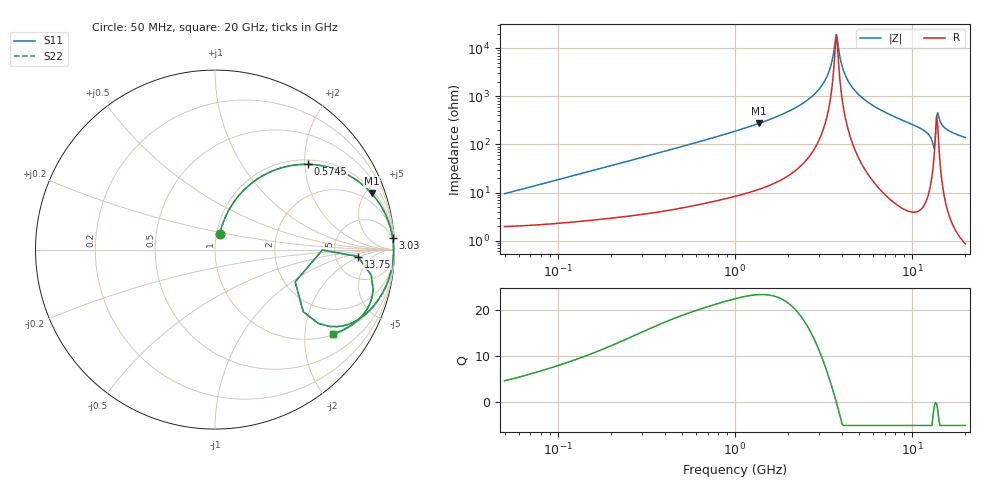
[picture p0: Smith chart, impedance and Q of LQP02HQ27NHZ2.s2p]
!Murata Part Number: LQP02HQ27NHZ2
!These Parameters are Measured in Series Mode Connection
!  o--[Z]--o
!Port1  Port2
!  o-------o
!Freq. Start=50[MHz] Stop=20[GHz], 401[Steps]
# Hz S RI R 50
!Freq.(Hz) S11(Real) S11(Imag) S21(Real) S21(Imag) S12(Real) S12(Imag) S22(Real) S22(Imag)
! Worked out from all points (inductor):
!   401 points, 50 MHz to 20 GHz, reference 50 ohm
!   read as one part in series: L = 29.4 nH near 51.52 MHz
!   highest Q = 23.4 at 1.37 GHz (marker M1), where L = 31.9 nH
!   self-resonance near 3.736 GHz
!   S11 on the Smith chart (normalised r, x): 50 MHz: 1.04, +0.19; 574.5 MHz: 1.11, +2.08; 3.03 GHz: 4, +30; 13.75 GHz: 8.53, -1.84; 20 GHz: 1.02, -2.77
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5e7  0.0273 0.0884  0.9727 -0.0884  0.9727 -0.0884  0.0273 0.0884
1.364002e8  0.079 0.2235  0.921 -0.2235  0.921 -0.2235  0.079 0.2235
3.721004e8  0.3201 0.4379  0.6799 -0.4379  0.6799 -0.4379  0.3201 0.4379
5.745257e8  0.5188 0.4749  0.4812 -0.4749  0.4812 -0.4749  0.5188 0.4749
1e9  0.7697 0.3994  0.2303 -0.3994  0.2303 -0.3994  0.7697 0.3994
1.369645e9  0.8727 0.3127  0.1273 -0.3127  0.1273 -0.3127  0.8727 0.3127
2.05233e9  0.9544 0.1864  0.0456 -0.1864  0.0456 -0.1864  0.9544 0.1864
2.728004e9  0.9836 0.0973  0.0164 -0.0973  0.0164 -0.0973  0.9836 0.0973
3.029571e9  0.9896 0.0648  0.0104 -0.0648  0.0104 -0.0648  0.9896 0.0648
3.364474e9  0.9933 0.0325  0.00666 -0.0325  0.00666 -0.0325  0.9933 0.0325
3.736399e9  0.9948 0.000128  0.00517 -0.000128  0.00517 -0.000128  0.9948 0.000128
3.850025e9  0.9949 -0.00913  0.00515 0.00913  0.00515 0.00913  0.9949 -0.00913
4.149438e9  0.9941 -0.0324  0.00588 0.0324  0.00588 0.0324  0.9941 -0.0324
4.608136e9  0.9912 -0.0651  0.00884 0.0651  0.00884 0.0651  0.9912 -0.0651
5.598765e9  0.9792 -0.1274  0.0208 0.1274  0.0208 0.1274  0.9792 -0.1274
7.442007e9  0.9431 -0.223  0.0569 0.223  0.0569 0.223  0.9431 -0.223
1.131968e10  0.8084 -0.3827  0.1916 0.3827  0.1916 0.3827  0.8084 -0.3827
1.295331e10  0.574 -0.4102  0.426 0.4102  0.426 0.4102  0.574 -0.4102
1.375312e10  0.7977 -0.0391  0.2023 0.0391  0.2023 0.0391  0.7977 -0.0391
1.438523e10  0.8733 -0.2718  0.1267 0.2718  0.1267 0.2718  0.8733 -0.2718
1.573793e10  0.8003 -0.3884  0.1997 0.3884  0.1997 0.3884  0.8003 -0.3884
2e10  0.6572 -0.4716  0.3428 0.4716  0.3428 0.4716  0.6572 -0.4716
